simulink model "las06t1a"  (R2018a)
settings: Solver=ode45  StartTime=0.0  StopTime=10  MaxStep=10  MinStep=0.0001  RelTol=1e-3  AbsTol=1e-3  EnableMultiTasking=on

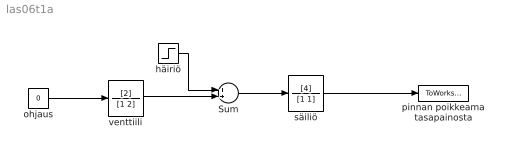
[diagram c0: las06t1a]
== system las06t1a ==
  Sum : Sum
  häiriö : Step  Time=3  After=-1
  ohjaus : Constant  Value=0
  pinnan poikkeama tasapainosta : ToWorkspace  VariableName=dh
  säiliö : TransferFcn  Numerator=[4]  Denominator=[1 1]
  venttiili : TransferFcn  Numerator=[2]  Denominator=[1 2]
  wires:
  häiriö/1 -> Sum/1
  venttiili/1 -> Sum/2
  Sum/1 -> säiliö/1
  säiliö/1 -> pinnan poikkeama tasapainosta/1
  ohjaus/1 -> venttiili/1
